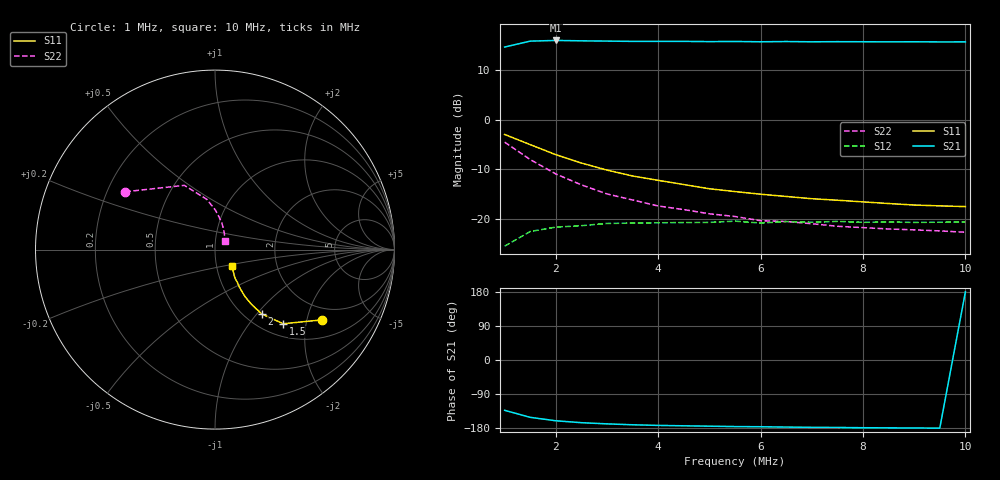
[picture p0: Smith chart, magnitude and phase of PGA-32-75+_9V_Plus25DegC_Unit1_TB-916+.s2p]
!Mini-Circuits Laboratory
!S-Parameters
!Model: PGA-32-75+
!Run / Lot / Date Code: N/A / CP621-001-03-01EV / N/A
!Fixture:
!Network Analyzer: PNA-X N5244A - 423 4 ports;  Serial number: 74314
!Date: 7/24/2017 at 7:48:21 AM
!S/N: Unit# 1
!Tested with:
# Hz  S  dB  R  50
!Frequency  S11 dB  S11 Deg  S21 dB  S21 Deg  S12 dB  S12 Deg  S22 dB  S22 Deg
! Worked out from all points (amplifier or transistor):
!   19 points, 1 MHz to 10 MHz, reference 50 ohm
!   highest |S21| = 16.0 dB at 2 MHz (marker M1)
!   |S21| within 3 dB of that: start of sweep to end of sweep
!   unconditionally stable (mu >= 1): start of sweep to end of sweep
!   at 2.5 MHz: K = 1.12, MAG = 16.6 dB, |S12| = -21.4 dB
!   at 5.5 MHz: K = 1.13, MAG = 16.0 dB, |S12| = -20.5 dB
!   at 10 MHz: K = 1.15, MAG = 15.8 dB, |S12| = -20.7 dB
!   S11 on the Smith chart (normalised r, x): 1 MHz: 1.55, -2.46; 1.5 MHz: 1.23, -1.49; 2 MHz: 1.19, -1.06; 10 MHz: 1.19, -0.22
1000000  -2.96 -33.4  14.69 -132.7  -25.53 86.9  -4.52 147.2
1500000  -5.02 -47.4  15.89 -151.3  -22.57 60.9  -8.03 115.5
2000000  -7.05 -54.0  16.02 -160.3  -21.68 45.6  -10.95 99.2
2500000  -8.74 -56.3  15.95 -165.5  -21.40 34.6  -13.15 89.4
3000000  -10.16 -57.4  15.89 -168.6  -20.94 30.4  -14.99 81.9
3500000  -11.36 -57.2  15.84 -171.0  -20.87 25.1  -16.20 76.0
4000000  -12.24 -56.8  15.84 -172.6  -20.81 22.2  -17.42 70.8
4500000  -13.08 -55.8  15.83 -173.6  -20.77 19.6  -18.14 66.9
5000000  -13.93 -55.3  15.79 -174.7  -20.73 15.9  -19.00 63.7
5500000  -14.51 -54.3  15.82 -175.7  -20.48 14.8  -19.54 60.3
6000000  -15.04 -53.1  15.75 -176.1  -20.87 13.9  -20.39 56.5
6500000  -15.49 -51.6  15.81 -177.0  -20.57 12.8  -20.55 54.6
7000000  -15.95 -50.4  15.75 -177.7  -20.70 10.2  -21.00 51.6
7500000  -16.25 -49.4  15.78 -178.1  -20.53 10.0  -21.52 48.2
8000000  -16.59 -48.4  15.76 -178.7  -20.72 8.6  -21.79 46.3
8500000  -16.92 -46.8  15.74 -179.0  -20.66 8.8  -22.06 45.1
9000000  -17.22 -46.0  15.76 -179.4  -20.73 6.9  -22.24 43.1
9500000  -17.40 -45.0  15.73 -179.8  -20.70 6.8  -22.45 39.6
1e7  -17.54 -44.2  15.74 179.9  -20.65 6.2  -22.72 38.2
